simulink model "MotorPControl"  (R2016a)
settings: Solver=VariableStepAuto  StartTime=0.0  StopTime=Tf  RelTol=1e-7  AbsTol=1e-6
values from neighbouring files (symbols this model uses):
  d = 0    [Section4p2_DCMotorOpenLoop.m]    (also in Section4p3_DCMotorPControl.m; Section4p4_DCMotorPIControl.m; Section4p5_RocketPDControl.m = -0.01; Section4p6_PIDSecondOrder.m = 2)
  Gden = [1 a0]    [Section4p2_DCMotorOpenLoop.m]    (also in Section4p3_DCMotorPControl.m = [J*L (J*R+b*L) (Kt*Ke+b*R)]; Section4p4_DCMotorPIControl.m; Section4p5_RocketPDControl.m = [1 a1 a0]; Section4p6_PIDSecondOrder.m = [1 a1 a0])
  Gnum = b0    (= 766.8)    [Section4p2_DCMotorOpenLoop.m]    (also in Section4p3_DCMotorPControl.m = 0.00122680374957; Section4p4_DCMotorPIControl.m; Section4p5_RocketPDControl.m = 6.32; Section4p6_PIDSecondOrder.m = 17)
  Kp = 16    [Section4p3_DCMotorPControl.m]    (also in Section4p4_DCMotorPIControl.m = 0.002; Section4p5_RocketPDControl.m = (wn^2-a0)/b0; Section4p6_PIDSecondOrder.m = 4.94237695078; Section4p6_PIFirstOrder.m = 2)
  r = 1000    [Section4p2_DCMotorOpenLoop.m]    (also in Section4p3_DCMotorPControl.m; Section4p4_DCMotorPIControl.m; Section4p5_RocketPDControl.m = 0.1; Section4p6_PIDSecondOrder.m = 4)
  Tf = 5    [Section4p2_DCMotorOpenLoop.m]    (also in Section4p3_DCMotorPControl.m = 0.005; Section4p4_DCMotorPIControl.m = 10; Section4p5_RocketPDControl.m = 10; Section4p6_PIDSecondOrder.m = 4)
  ulim = inf    [Section4p3_DCMotorPControl.m]    (also in Section4p4_DCMotorPIControl.m; Section4p5_RocketPDControl.m)

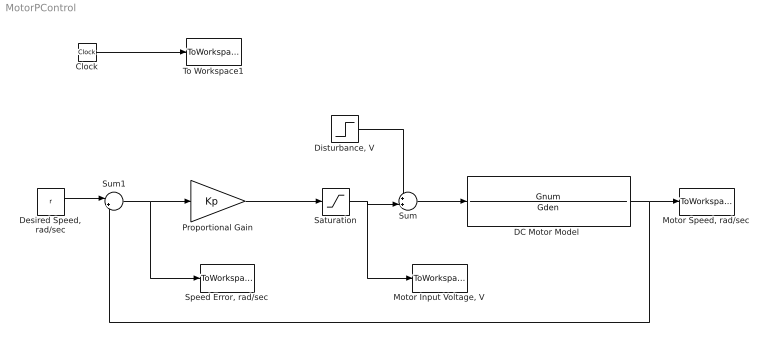
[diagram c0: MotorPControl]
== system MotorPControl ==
  Clock : Clock
  "DC Motor Model " : TransferFcn  Numerator=Gnum  Denominator=Gden
  "Desired Speed, rad/sec" : Constant  Value=r
  "Disturbance, V" : Step  Time=Tf/2  After=d  SampleTime=0
  "Motor Input Voltage, V" : ToWorkspace  VariableName=u  SampleTime=-1
  "Motor Speed, rad/sec" : ToWorkspace  VariableName=y  SampleTime=-1
  Proportional Gain : Gain  Gain=Kp
  Saturation : Saturate  UpperLimit=ulim  LowerLimit=-ulim
  "Speed Error, rad/sec" : ToWorkspace  VariableName=e  SampleTime=-1
  Sum : Sum  Inputs=++|
  Sum1 : Sum  Inputs=|+-
  To Workspace1 : ToWorkspace  VariableName=t  SampleTime=-1
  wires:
  Clock/1 -> To Workspace1/1
  "Disturbance, V"/1 -> Sum/1
  Proportional Gain/1 -> Saturation/1
  Sum/1 -> "DC Motor Model "/1
  "DC Motor Model "/1 -> Sum1/2, "Motor Speed, rad/sec"/1
  "Desired Speed, rad/sec"/1 -> Sum1/1
  Sum1/1 -> Proportional Gain/1, "Speed Error, rad/sec"/1
  Saturation/1 -> Sum/2, "Motor Input Voltage, V"/1
